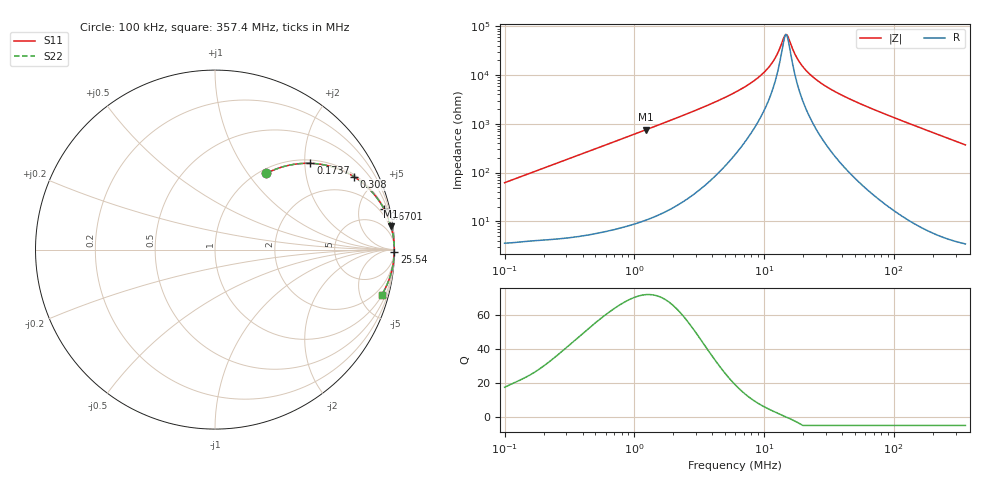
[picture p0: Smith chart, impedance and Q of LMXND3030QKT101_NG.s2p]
! LMXND3030QKT101_NG  S-PARAMETER MODEL  ( Standard Model )
! Model Generated by TAIYO YUDEN Corporation (https://www.yuden.co.jp/en/)
! Version 1.0
! TAIYO YUDEN Control No. 20250925
! Copyright(c) 2025 TAIYO YUDEN CO.,LTD. All Rights Reserved.
! Product Description (link to TY-COMPAS)
! https://ds.yuden.co.jp/TYCOMPAS/or/detail?pn=LMXND3030QKT101MNG&u=M
! Products Name : Inductors
! Characteristics :
!  Inductance : 100 [uH] , SRF(min) : 7.0 [MHz] , DC Resistance(max) : 2.88 [Ohm]
!  Rated Current : Saturation  230 [mA] , Temp Rise  230 [mA] (40 [degC])
!  Case Size : 3.0 x 3.0 / 0.118 x 0.118 [mm/inch] , Thickness : 1.5 / 0.059 [mm/inch]
!  (Conditions: Temperature = 25 [degC] , DC Bias Current = 0 [A])
! External Node Assignments :
!  1  o---GGG---o  2
! GND o---------o GND
! Frequency Range : 0.1MHz  -  357.398349MHz  [ 402 STEP ]
# MHz S RI R 50
! Freq[MHz].  S11 Real  S11 Imag  S21 Real  S21 Imag  S12 Real  S12 Imag  S22 Real  S22 Imag
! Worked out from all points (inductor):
!   401 points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, 100 kHz to 357.4 MHz, reference 50 ohm
!   read as one part in series: L = 98 uH near 104.2 kHz
!   highest Q = 71.8 at 1.238 MHz (marker M1), where L = 97.6 uH
!   self-resonance near 14.7 MHz
!   S11 on the Smith chart (normalised r, x): 100 kHz: 1.07, +1.23; 173.7 kHz: 1.08, +2.13; 308 kHz: 1.09, +3.77; 670.1 kHz: 1.13, +8.19; 25.54 MHz: open; 357.4 MHz: 1.07, -7.38
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0.1  0.2869 0.4246  0.7131 -0.4246  0.7131 -0.4246  0.2869 0.4246
0.173715  0.5313 0.4806  0.4687 -0.4806  0.4687 -0.4806  0.5313 0.4806
0.308006  0.775 0.4057  0.225 -0.4057  0.225 -0.4057  0.775 0.4057
0.393689  0.8479 0.349  0.1521 -0.349  0.1521 -0.349  0.8479 0.349
0.670051  0.9405 0.2287  0.0595 -0.2287  0.0595 -0.2287  0.9405 0.2287
1.23764  0.9812 0.129  0.0188 -0.129  0.0188 -0.129  0.9812 0.129
1.549909  0.9877 0.1033  0.0123 -0.1033  0.0123 -0.1033  0.9877 0.1033
3.585124  0.9971 0.0427  0.00288 -0.0427  0.00288 -0.0427  0.9971 0.0427
6.101817  0.9983 0.0219  0.00168 -0.0219  0.00168 -0.0219  0.9983 0.0219
8.464187  0.9985 0.0127  0.00153 -0.0127  0.00153 -0.0127  0.9985 0.0127
10.59978  0.9985 0.00732  0.00151 -0.00732  0.00151 -0.00732  0.9985 0.00732
12.23143  0.9985 0.00413  0.00149 -0.00413  0.00149 -0.00413  0.9985 0.00413
14.11423  0.9985 0.00103  0.00146 -0.00103  0.00146 -0.00103  0.9985 0.00103
14.70358  0.9985 0.000145  0.00145 -0.000145  0.00145 -0.000145  0.9985 0.000145
15.31753  0.9986 -0.000738  0.00144 0.000738  0.00144 0.000738  0.9986 -0.000738
17.31754  0.9986 -0.00341  0.0014 0.00341  0.0014 0.00341  0.9986 -0.00341
18.79393  0.9986 -0.00523  0.00138 0.00523  0.00138 0.00523  0.9986 -0.00523
23.53582  0.9987 -0.0105  0.00133 0.0105  0.00133 0.0105  0.9987 -0.0105
25.54235  0.9987 -0.0126  0.00133 0.0126  0.00133 0.0126  0.9987 -0.0126
41.73016  0.9983 -0.0273  0.00171 0.0273  0.00171 0.0273  0.9983 -0.0273
92.65788  0.9945 -0.068  0.00554 0.068  0.00554 0.068  0.9945 -0.068
357.3983  0.9296 -0.2512  0.0704 0.2512  0.0704 0.2512  0.9296 -0.2512
